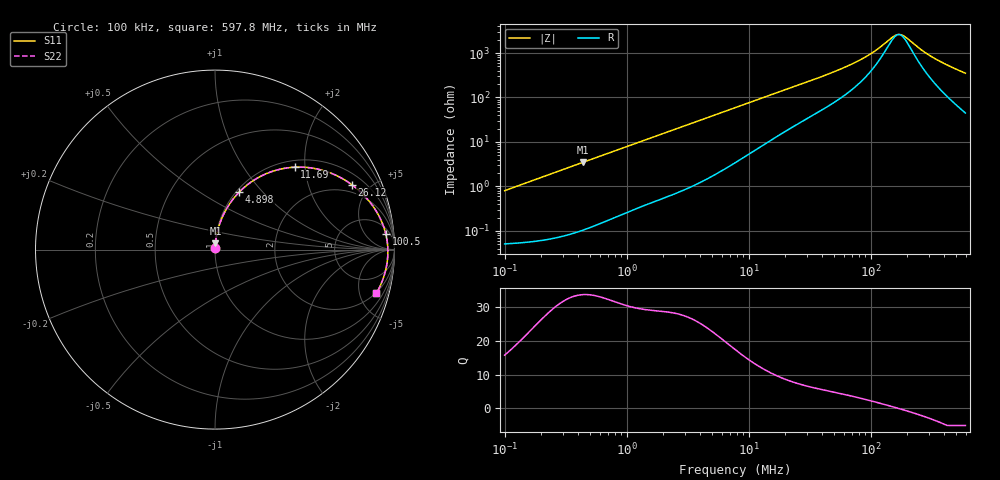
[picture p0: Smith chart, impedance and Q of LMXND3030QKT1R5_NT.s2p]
! LMXND3030QKT1R5_NT  S-PARAMETER MODEL  ( Standard Model )
! Model Generated by TAIYO YUDEN Corporation (https://www.yuden.co.jp/en/)
! Version 1.0
! TAIYO YUDEN Control No. 20250925
! Copyright(c) 2025 TAIYO YUDEN CO.,LTD. All Rights Reserved.
! Product Description (link to TY-COMPAS)
! https://ds.yuden.co.jp/TYCOMPAS/or/detail?pn=LMXND3030QKT1R5NNT&u=M
! Products Name : Inductors
! Characteristics :
!  Inductance : 1.5 [uH] , SRF(min) : 87 [MHz] , DC Resistance(max) : 0.046 [Ohm]
!  Rated Current : Saturation  1800 [mA] , Temp Rise  2800 [mA] (40 [degC])
!  Case Size : 3.0 x 3.0 / 0.118 x 0.118 [mm/inch] , Thickness : 1.5 / 0.059 [mm/inch]
!  (Conditions: Temperature = 25 [degC] , DC Bias Current = 0 [A])
! External Node Assignments :
!  1  o---GGG---o  2
! GND o---------o GND
! Frequency Range : 0.1MHz  -  597.797849MHz  [ 402 STEP ]
# MHz S RI R 50
! Freq[MHz].  S11 Real  S11 Imag  S21 Real  S21 Imag  S12 Real  S12 Imag  S22 Real  S22 Imag
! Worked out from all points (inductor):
!   401 points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, 100 kHz to 597.8 MHz, reference 50 ohm
!   read as one part in series: L = 1.27 uH near 104.4 kHz
!   highest Q = 33.5 at 438.5 kHz (marker M1), where L = 1.27 uH
!   self-resonance near 169.9 MHz
!   S11 on the Smith chart (normalised r, x): 100 kHz: 1.00, +0.02; 4.898 MHz: 1.03, +0.75; 11.69 MHz: 1.14, +1.77; 26.12 MHz: 1.53, +3.85; 100.5 MHz: 9, +18; 597.8 MHz: 1.90, -6.97
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0.1  0.000574 0.00801  0.9994 -0.00801  0.9994 -0.00801  0.000574 0.00801
0.429114  0.00218 0.034  0.9978 -0.034  0.9978 -0.034  0.00218 0.034
0.438545  0.00225 0.0348  0.9978 -0.0348  0.9978 -0.0348  0.00225 0.0348
0.959189  0.00808 0.0746  0.9919 -0.0746  0.9919 -0.0746  0.00808 0.0746
1.84139  0.0247 0.1386  0.9753 -0.1386  0.9753 -0.1386  0.0247 0.1386
3.170884  0.0637 0.2264  0.9363 -0.2264  0.9363 -0.2264  0.0637 0.2264
4.897879  0.1341 0.3197  0.8659 -0.3197  0.8659 -0.3197  0.1341 0.3197
7.731739  0.27 0.4161  0.73 -0.4161  0.73 -0.4161  0.27 0.4161
11.68594  0.4444 0.4593  0.5556 -0.4593  0.5556 -0.4593  0.4444 0.4593
16.91091  0.6073 0.4394  0.3927 -0.4394  0.3927 -0.4394  0.6073 0.4394
26.1213  0.7611 0.3625  0.2389 -0.3625  0.2389 -0.3625  0.7611 0.3625
33.17799  0.8223 0.3102  0.1777 -0.3102  0.1777 -0.3102  0.8223 0.3102
62.32327  0.9198 0.175  0.0802 -0.175  0.0802 -0.175  0.9198 0.175
100.5451  0.9519 0.0863  0.0481 -0.0863  0.0481 -0.0863  0.9519 0.0863
142.3714  0.9614 0.0285  0.0386 -0.0285  0.0386 -0.0285  0.9614 0.0285
162.2076  0.9629 0.00743  0.0371 -0.00743  0.0371 -0.00743  0.9629 0.00743
180.8332  0.9632 -0.0101  0.0368 0.0101  0.0368 0.0101  0.9632 -0.0101
197.2621  0.963 -0.0242  0.037 0.0242  0.037 0.0242  0.963 -0.0242
261.6867  0.9589 -0.0717  0.0411 0.0717  0.0411 0.0717  0.9589 -0.0717
318.2396  0.9525 -0.1072  0.0475 0.1072  0.0475 0.1072  0.9525 -0.1072
431.4531  0.9344 -0.1687  0.0656 0.1687  0.0656 0.1687  0.9344 -0.1687
597.7978  0.8984 -0.2446  0.1016 0.2446  0.1016 0.2446  0.8984 -0.2446
